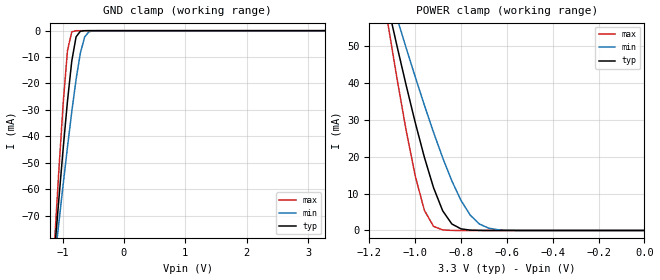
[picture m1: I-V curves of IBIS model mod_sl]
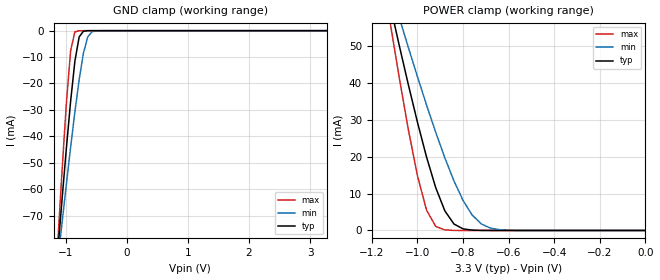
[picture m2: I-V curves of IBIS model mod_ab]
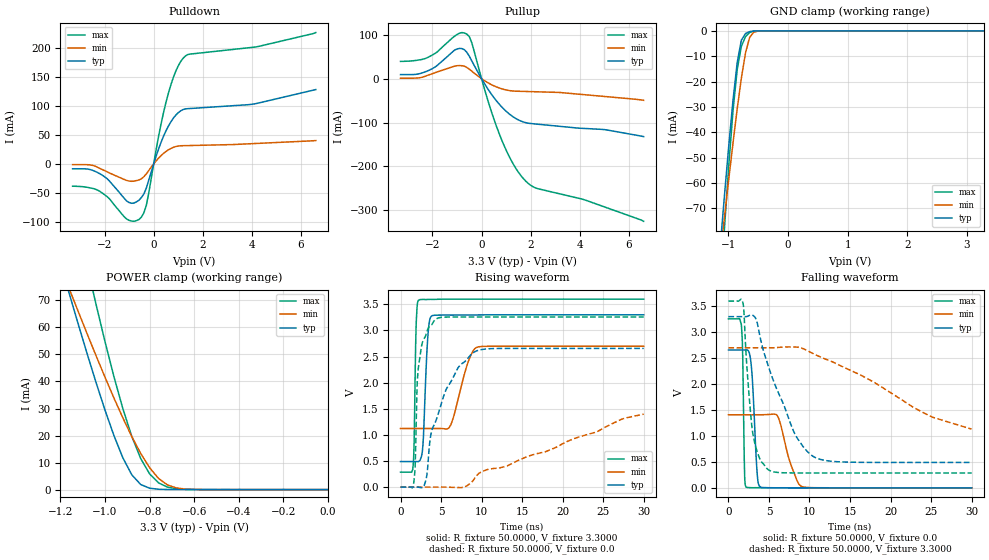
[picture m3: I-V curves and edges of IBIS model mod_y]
| IBIS (I/O, Buffer, Information, Specification) Model, officially
| electronic behavioral standard for Buffer structures of digital pins.
[IBIS ver]  4.0
[File name] 54ac157_3v3_rev1.ibs
[File Rev]  1.0
[Date]   7 Sep 2018
[Source]   CAD & Design Services (Catania) - STMicroelectronics
[Notes]
  (Note1) This IBIS model is the model of the product with package
   (Flat16 package elements);
  (Note2) This IBIS model is extracted with nominal 3.3V power supply
   (min:3.0V, typ:3.3V, max:3.6V);
  (Note3) This model has few Warnings about the non-monotonicity
   of I-V curves, but they are not indicative of problems
   inside the model;
[Copyright] (c) 2018 STMicroelectronics
|   Component 54AC157
[Component] RHF54AC157
[Manufacturer] STMicroelectronics
[Package]
| variable  typ   min   max
R_pkg   0.0   0.0   0.0
L_pkg   0.0H   0.0H   0.0H
C_pkg   0.0F   0.0F   0.0F
[Pin]   signal_name   model_name   R_pin   L_pin   C_pin
1   SELECT   mod_sl   87.8m   2.68nH   1.16pF
2   1A   mod_ab   53.6m   1.94nH   1.11pF
3   1B   mod_ab   34.1m   1.02nH   0.87pF
4   1Y   mod_y   34.1m   1.02nH   0.87pF
5   2A   mod_ab   34.1m   1.02nH   0.87pF
6   2B   mod_ab   34.1m   1.02nH   0.87pF
7   2Y   mod_y   53.6m   1.94nH   1.11pF
8   GND   GND   87.8m   2.68nH   1.16pF
9   3Y   mod_y   87.8m   2.68nH   1.16pF
10   3B   mod_ab   53.6m   1.94nH   1.11pF
11   3A   mod_ab   34.1m   1.02nH   0.87pF
12   4Y   mod_y   34.1m   1.02nH   0.87pF
13   4B   mod_ab   34.1m   1.02nH   0.87pF
14   4A   mod_ab   34.1m   1.02nH   0.87pF
15   STROB   mod_sl   53.6m   1.94nH   1.11pF
16   VCC   POWER   87.8m   2.68nH   1.16pF
| Models and submodels in the file (3): mod_sl (Input), mod_ab (Input), mod_y (I/O)
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|   Model mod_sl
[Model]   mod_sl
Model_type Input
Vinl   =   0.800V
Vinh   =   2.000V
C_comp   0.532pF   0.485pF   0.611pF
[Temperature Range]  25.0000   0.1250k   -55.0000
[Voltage Range]   3.3000V   2.7000V   3.6000V
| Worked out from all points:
|   GND clamp passes 1 mA (typ) near -0.74 V on its own axis
|   POWER clamp passes 1 mA (typ) near -0.82 V on its own axis
[GND_clamp]
|Voltage   I(typ)   I(min)   I(max)
-3.3V     -748.7mA   -577.4mA   -1.01A
-1.13V    -83.56mA   -87.5mA    -80.12mA
-1.06V    -63.73mA   -72.7mA    -52.87mA
-990mV    -44.59mA   -58.19mA   -27.57mA
-920mV    -26.71mA   -44.12mA   -7.572mA
-850mV    -11.51mA   -30.73mA   -438.3uA
-780mV    -2.357mA   -18.5mA    -11.16uA
-710mV    -202.6uA   -8.472mA   -269.9nA
-640mV    -13.61uA   -2.375mA   -6.525nA
-570mV    -893.7nA   -396.9uA   -166.8pA
-430mV    -3.851nA   -7.049uA   -9.012pA
3.28V     6.52pA     37.08uA    5.92pA
[POWER_clamp]
|Voltage   I(typ)   I(min)   I(max)
-3.28V    720.8mA    551.4mA    979.5mA
-1.12V    61.06mA    65.83mA    56.34mA
-1.08V    50.08mA    57.6mA     41.36mA
-1.04V    39.43mA    49.5mA     27.27mA
-1V       29.26mA    41.59mA    14.79mA
-960mV    19.82mA    33.91mA    5.475mA
-920mV    11.59mA    26.56mA    1.113mA
-880mV    5.322mA    19.66mA    149.4uA
-840mV    1.751mA    13.42mA    18.09uA
-760mV    95.85uA    4.17mA     257.2nA
-680mV    4.309uA    633.7uA    3.657nA
0V        6.6pA      43.3pA     7.2pA
|   Model mod_ab
[Model]   mod_ab
Model_type Input
Vinl   =   0.800V
Vinh   =   2.000V
C_comp   0.584pF   0.423pF   0.769pF
[Temperature Range]  25.0000   0.1250k   -55.0000
[Voltage Range]   3.3000V   2.7000V   3.6000V
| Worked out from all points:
|   GND clamp passes 1 mA (typ) near -0.74 V on its own axis
|   POWER clamp passes 1 mA (typ) near -0.82 V on its own axis
[GND_clamp]
|Voltage   I(typ)   I(min)   I(max)
-3.3V     -748.7mA   -577.4mA   -1.01A
-1.13V    -83.56mA   -87.5mA    -80.12mA
-1.06V    -63.73mA   -72.7mA    -52.87mA
-990mV    -44.59mA   -58.19mA   -27.57mA
-920mV    -26.71mA   -44.12mA   -7.572mA
-850mV    -11.51mA   -30.73mA   -438.3uA
-780mV    -2.357mA   -18.5mA    -11.16uA
-710mV    -202.6uA   -8.472mA   -269.9nA
-640mV    -13.61uA   -2.375mA   -6.525nA
-570mV    -893.7nA   -396.9uA   -166.8pA
-430mV    -3.851nA   -7.049uA   -9.012pA
3.28V     6.52pA     37.08uA    5.92pA
[POWER_clamp]
|Voltage   I(typ)   I(min)   I(max)
-3.28V    720.8mA    551.4mA    979.5mA
-1.12V    61.06mA    65.83mA    56.34mA
-1.08V    50.08mA    57.6mA     41.36mA
-1.04V    39.43mA    49.5mA     27.27mA
-1V       29.26mA    41.59mA    14.79mA
-960mV    19.82mA    33.91mA    5.475mA
-920mV    11.59mA    26.56mA    1.113mA
-880mV    5.322mA    19.66mA    149.4uA
-840mV    1.751mA    13.42mA    18.09uA
-760mV    95.85uA    4.17mA     257.2nA
-680mV    4.309uA    633.7uA    3.657nA
0V        6.6pA      43.3pA     7.2pA
|   Model mod_y
[Model]   mod_y
Model_type I/O
Polarity   Non-Inverting
Vinl   =  0.800V
Vinh   =  2.000V
Vmeas   =  1.650V
Cref   =  50pF
Rref   =  500
C_comp   3.207pF   2.324pF   4.228pF
[Temperature Range]  25.0000   0.1250k   -55.0000
[Voltage Range]   3.3000V   2.7000V   3.6000V
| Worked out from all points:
|   slope of the pulldown table from 0 to 0.495 V, typ, clamps not added: 8.73 ohm
|   slope of the pullup table from 0 to 0.495 V, typ, clamps not added: 11.6 ohm
|   GND clamp passes 1 mA (typ) near -0.71 V on its own axis
|   POWER clamp passes 1 mA (typ) near -0.81 V on its own axis
|   rising waveform, R_fixture 50.0000, V_fixture 3.3000: 20-80 % time 459ps typ, 1.61ns min, 213ps max; typ from 0.489 V to 3.3 V
|   rising waveform, R_fixture 50.0000, V_fixture 0.0: 20-80 % time 3.15ns typ, 15.1ns min, 648ps max; typ from 0 V to 2.66 V
|   falling waveform, R_fixture 50.0000, V_fixture 0.0: 20-80 % time 503ps typ, 1.52ns min, 193ps max; typ from 2.66 V to 0 V
|   falling waveform, R_fixture 50.0000, V_fixture 3.3000: 20-80 % time 4.01ns typ, 10.7ns min, 1.07ns max; typ from 3.3 V to 0.489 V
[Pulldown]
|Voltage   I(typ)   I(min)   I(max)
-3.3V     -8.332mA   -1.212mA   -38.54mA
-2.3V     -14.47mA   -5.536mA   -44.93mA
-1.9V     -25.37mA   -13.5mA    -56.42mA
-1.1V     -64.17mA   -28.57mA   -95.26mA
-600mV    -62.92mA   -27.78mA   -96.25mA
-300mV    -42.06mA   -17.27mA   -72.02mA
200mV     25.93mA    10.07mA    47.73mA
600mV     65.52mA    24.42mA    122.5mA
900mV     84.46mA    30.13mA    160.6mA
1.2V      94.2mA     31.63mA    183.1mA
4.1V      103.9mA    35.33mA    202.3mA
6.6V      128.8mA    40.53mA    227.5mA
[Pullup]
|Voltage   I(typ)   I(min)   I(max)
-3.3V     9.332mA    1.212mA    39.54mA
-2.2V     17.76mA    7.601mA    48.21mA
-1.1V     65.17mA    28.57mA    97.06mA
-600mV    60.24mA    25.52mA    101.7mA
-400mV    40.78mA    17.2mA     82.3mA
300mV     -27.16mA   -10.53mA   -57.61mA
800mV     -63.16mA   -22.72mA   -137.1mA
1.3V      -87.59mA   -28.2mA    -195.8mA
1.8V      -100.4mA   -29.15mA   -233.9mA
2.2V      -103.4mA   -29.79mA   -249.4mA
4.1V      -113.3mA   -36.05mA   -274.9mA
6.6V      -132.2mA   -49.33mA   -325.5mA
[GND_clamp]
|Voltage   I(typ)   I(min)   I(max)
-3.3V     -748.8mA   -577.4mA   -1.02A
-1.13V    -83.86mA   -87.56mA   -102.6mA
-1.06V    -64.09mA   -72.76mA   -76.81mA
-990mV    -45.06mA   -58.26mA   -52.71mA
-920mV    -27.37mA   -44.2mA    -31.5mA
-850mV    -12.5mA    -30.82mA   -15.3mA
-780mV    -3.656mA   -18.61mA   -6.086mA
-710mV    -1.018mA   -8.602mA   -2.236mA
-640mV    -262.4uA   -2.487mA   -621uA
-570mV    -57.31uA   -454.5uA   -83.06uA
-500mV    -11.95uA   -74.72uA   -9.782uA
3.28V     84.16pA    36.76uA    15.02pA
[POWER_clamp]
|Voltage   I(typ)   I(min)   I(max)
-3.28V    720.9mA    551.4mA    1.006A
-1.16V    72.37mA    74.17mA    112.6mA
-1.12V    61.16mA    65.81mA    97.5mA
-1.08V    50.19mA    57.57mA    82.74mA
-1.04V    39.55mA    49.48mA    68.43mA
-960mV    19.98mA    33.88mA    41.77mA
-880mV    5.49mA     19.63mA    19.69mA
-840mV    1.883mA    13.38mA    11.5mA
-800mV    511.9uA    8.091mA    5.814mA
-760mV    132.6uA    4.139mA    2.496mA
-640mV    3.963uA    205.7uA    111uA
0V        86.27pA    2.522nA    22.24pA
[Ramp]
| variable   typ   min   max
dV/dt_r  1.5938/3.1478n   0.6763/11.5077n   1.9546/0.6551n
dV/dt_f  1.6864/3.9992n   0.5092/10.6280n   1.9882/1.0836n
R_load = 50.0000
[Rising Waveform]
R_fixture= 50.0000
V_fixture= 3.3000
V_fixture_min= 2.7000
V_fixture_max= 3.6000
|time   V(typ)   V(min)   V(max)
0s        489.4mV    1.122V     286.6mV
1.56ns    489.4mV    1.122V     412.8mV
1.92ns    489.6mV    1.122V     3.06V
2.19ns    487.7mV    1.122V     3.575V
2.7ns     693.6mV    1.123V     3.594V
3.36ns    2.862V     1.123V     3.594V
3.84ns    3.277V     1.123V     3.595V
6.21ns    3.294V     1.195V     3.6V
9.39ns    3.297V     2.676V     3.6V
30ns      3.3V       2.699V     3.6V
[Rising Waveform]
R_fixture= 50.0000
V_fixture= 0.0
V_fixture_min= 0.0
V_fixture_max= 0.0
|time   V(typ)   V(min)   V(max)
0s        0V         0V         0V
1.59ns    -1.304uV   410.8nV    44.16mV
1.8ns     -18.3uV    59.3nV     379.1mV
2.04ns    509.1uV    -2.505uV   1.912V
2.22ns    -1.261mV   -1.652uV   2.305V
3.12ns    131.2mV    -347.8nV   2.91V
4.26ns    1.227V     -4.085uV   3.202V
7.08ns    2.282V     -7.735mV   3.258V
9.3ns     2.603V     205.5mV    3.258V
30ns      2.657V     1.398V     3.258V
[Falling Waveform]
R_fixture= 50.0000
V_fixture= 0.0
V_fixture_min= 0.0
V_fixture_max= 0.0
|time   V(typ)   V(min)   V(max)
0s        2.657V     1.408V     3.258V
1.59ns    2.656V     1.408V     3.149V
1.77ns    2.657V     1.408V     2.476V
2.01ns    2.658V     1.408V     176mV
2.19ns    2.66V      1.408V     12.07mV
2.79ns    2.401V     1.408V     3.408mV
3.57ns    227.3mV    1.408V     2.903mV
4.05ns    9.194mV    1.409V     1.974mV
8.97ns    1.66mV     30.19mV    10.05uV
30ns      -228.4nV   658.3uV    -921.6nV
[Falling Waveform]
R_fixture= 50.0000
V_fixture= 3.3000
V_fixture_min= 2.7000
V_fixture_max= 3.6000
|time   V(typ)   V(min)   V(max)
0s        3.3V       2.7V       3.6V
1.8ns     3.3V       2.7V       3.559V
2.34ns    3.305V     2.7V       2.196V
3ns       3.327V     2.7V       1.056V
3.9ns     2.911V     2.7V       549.2mV
4.92ns    2.347V     2.7V       349.6mV
8.22ns    1.032V     2.715V     287.3mV
10.8ns    577.7mV    2.561V     286.7mV
25.2ns    489.4mV    1.36V      286.6mV
30ns      489.4mV    1.133V     286.6mV
